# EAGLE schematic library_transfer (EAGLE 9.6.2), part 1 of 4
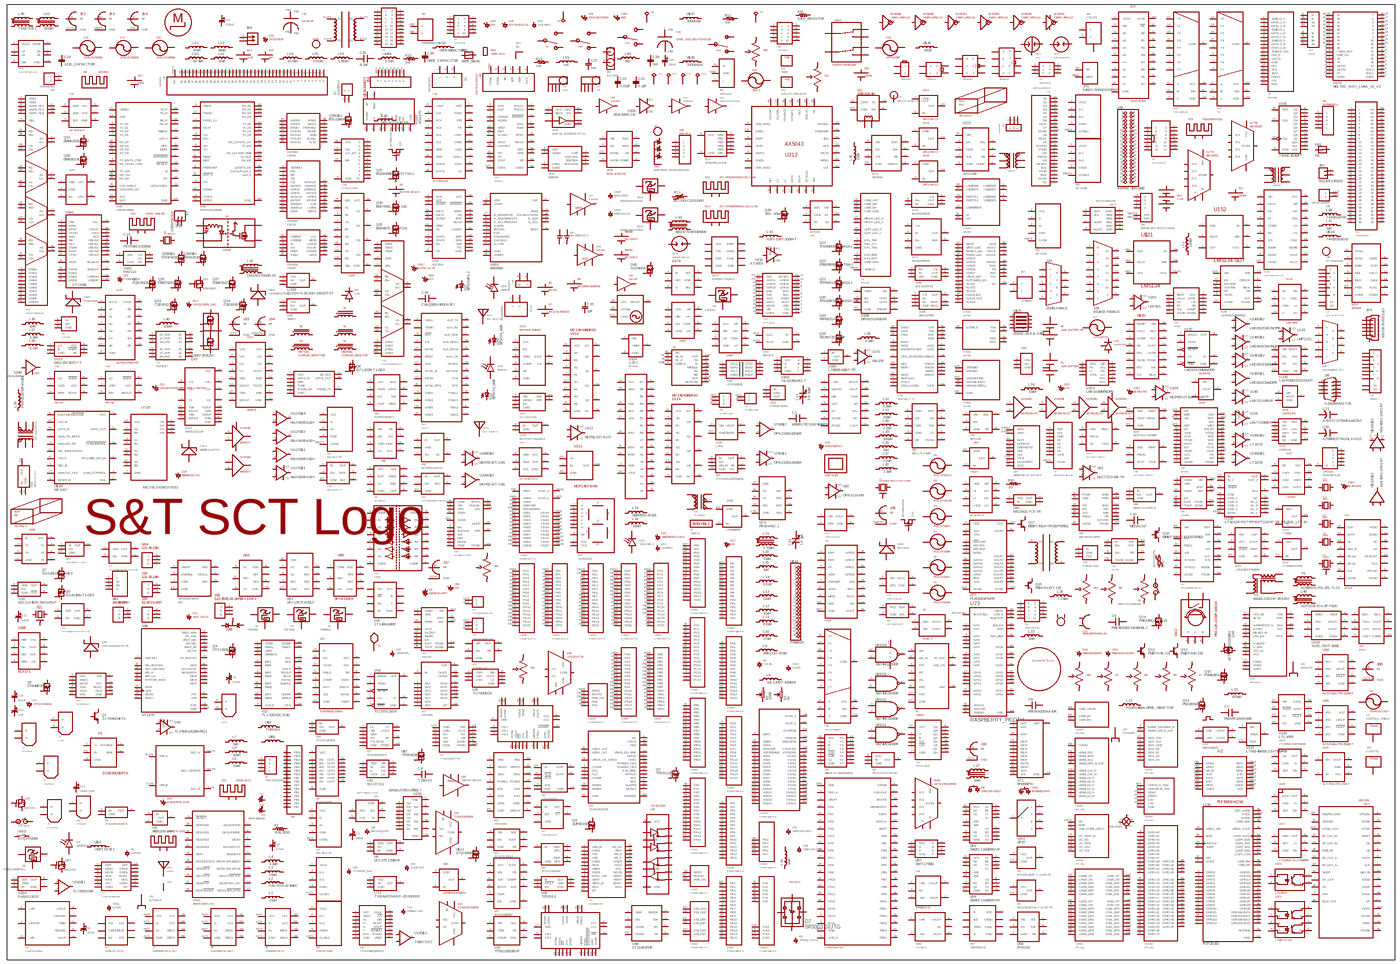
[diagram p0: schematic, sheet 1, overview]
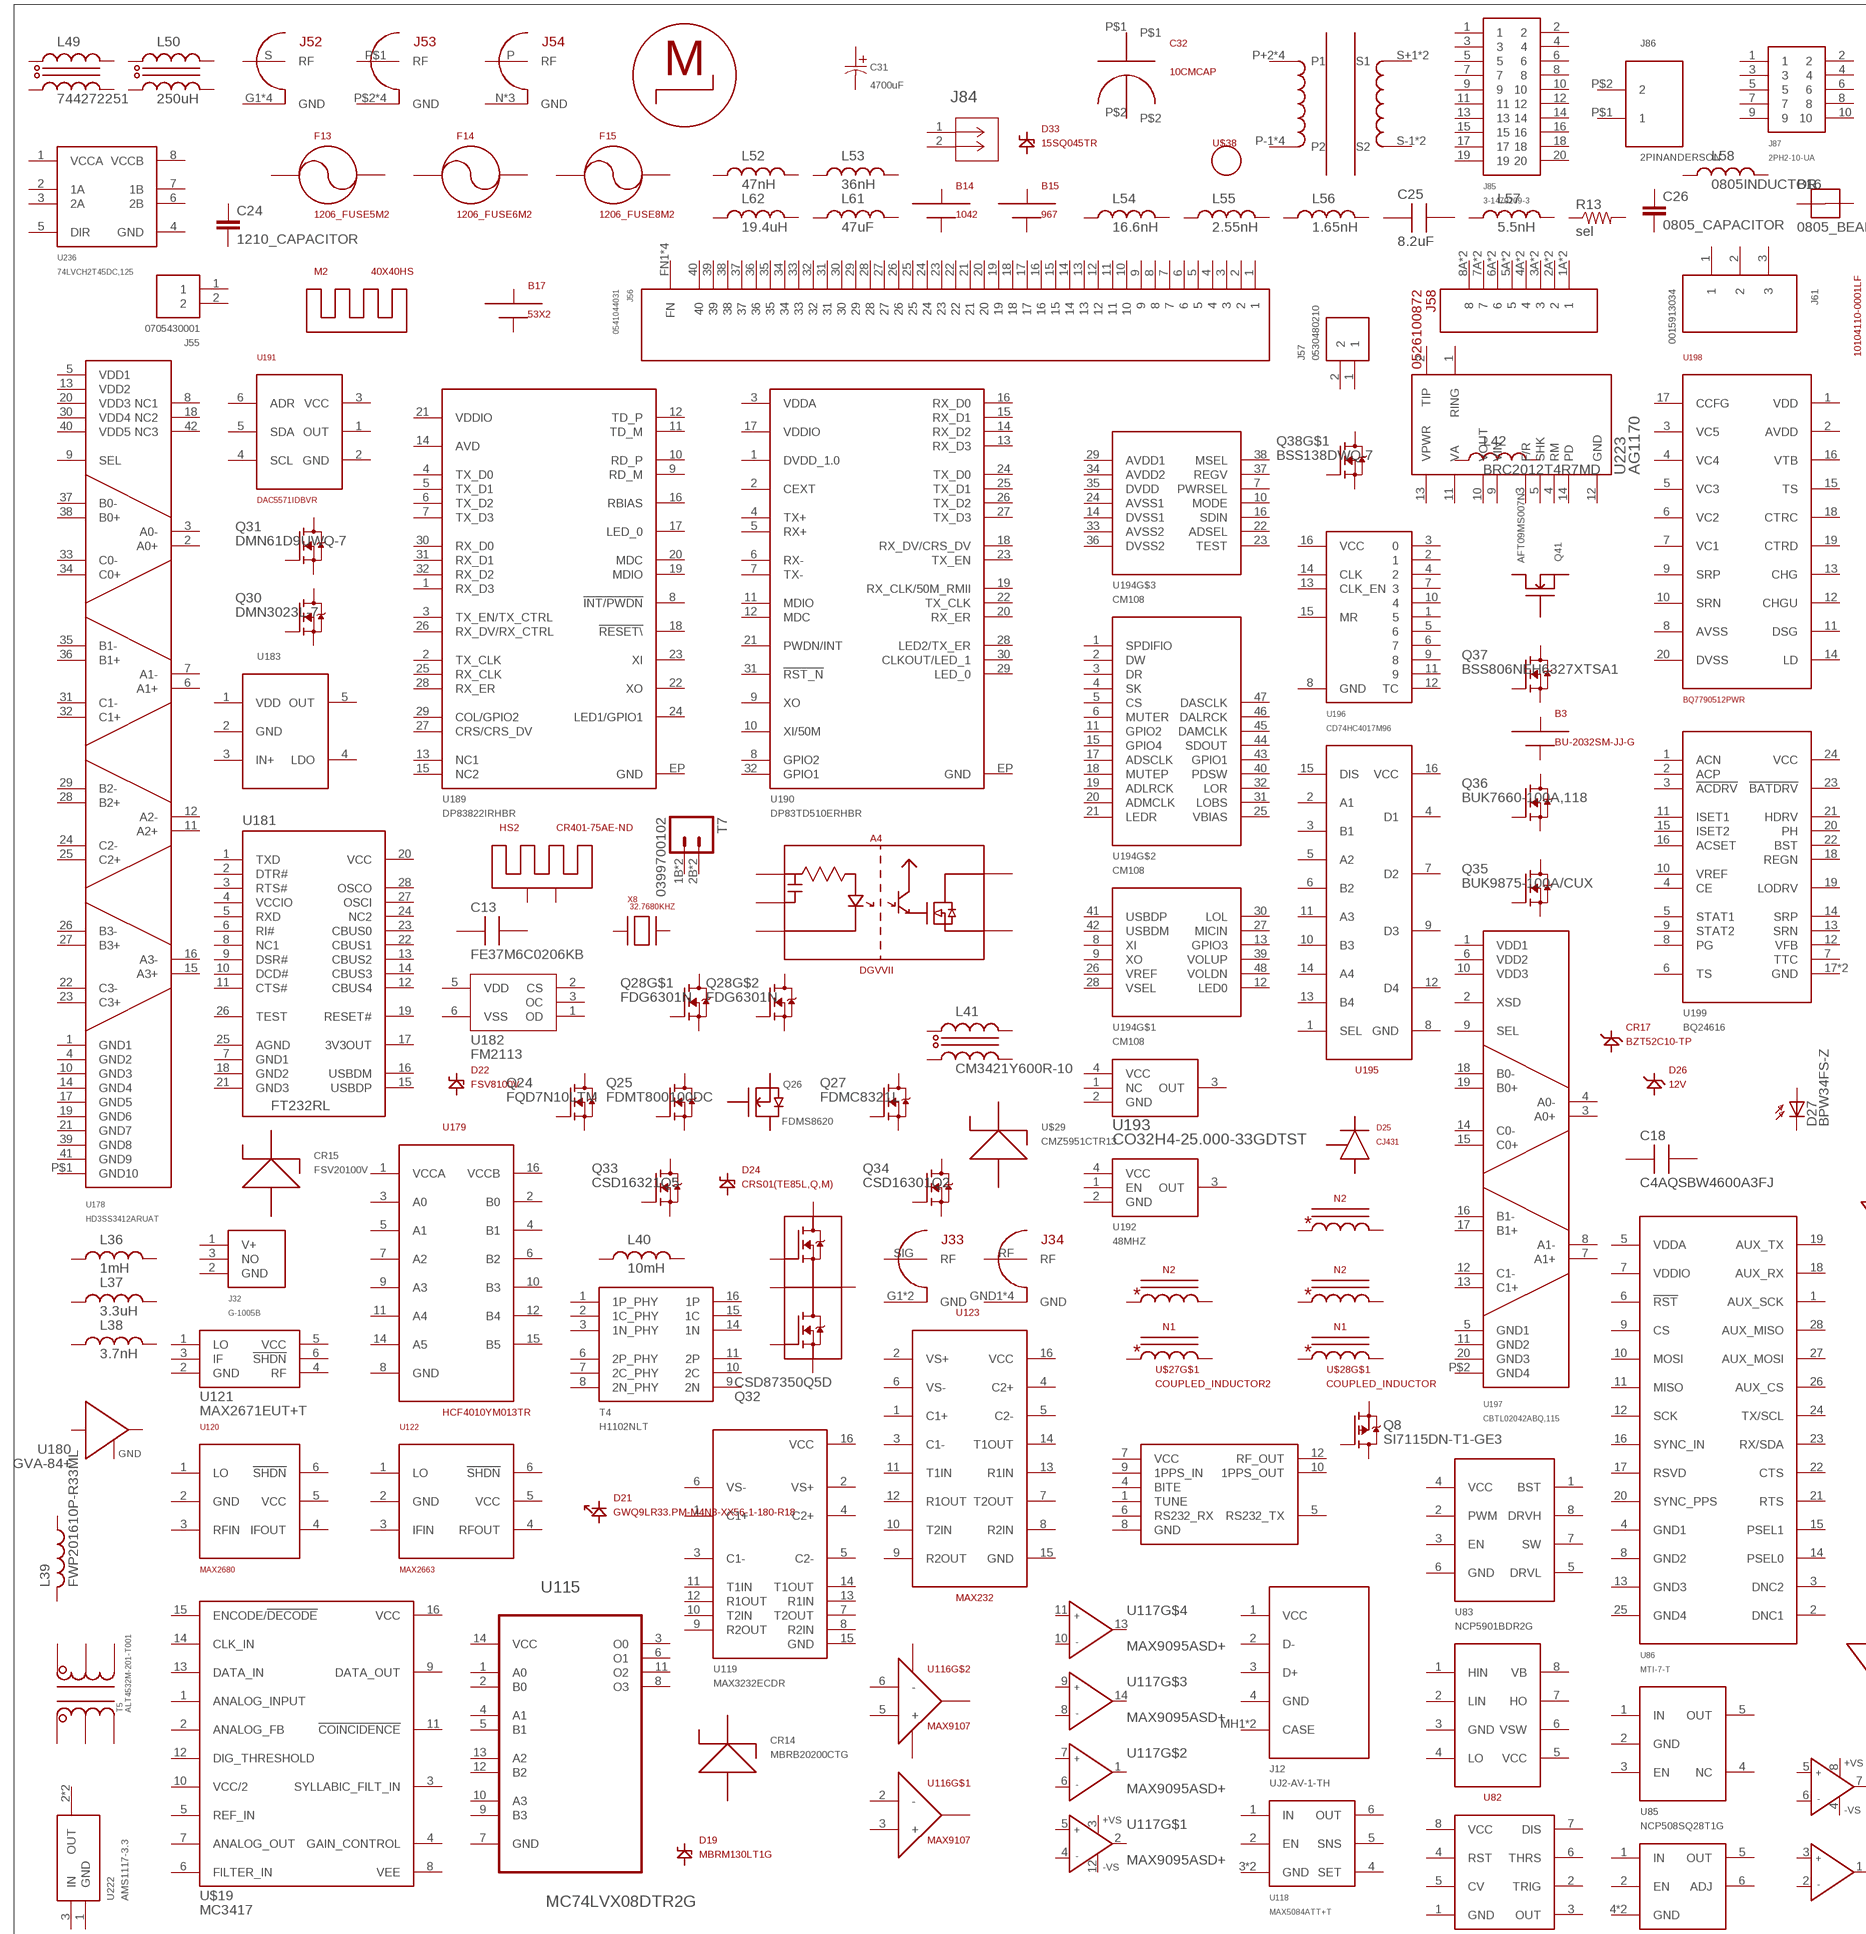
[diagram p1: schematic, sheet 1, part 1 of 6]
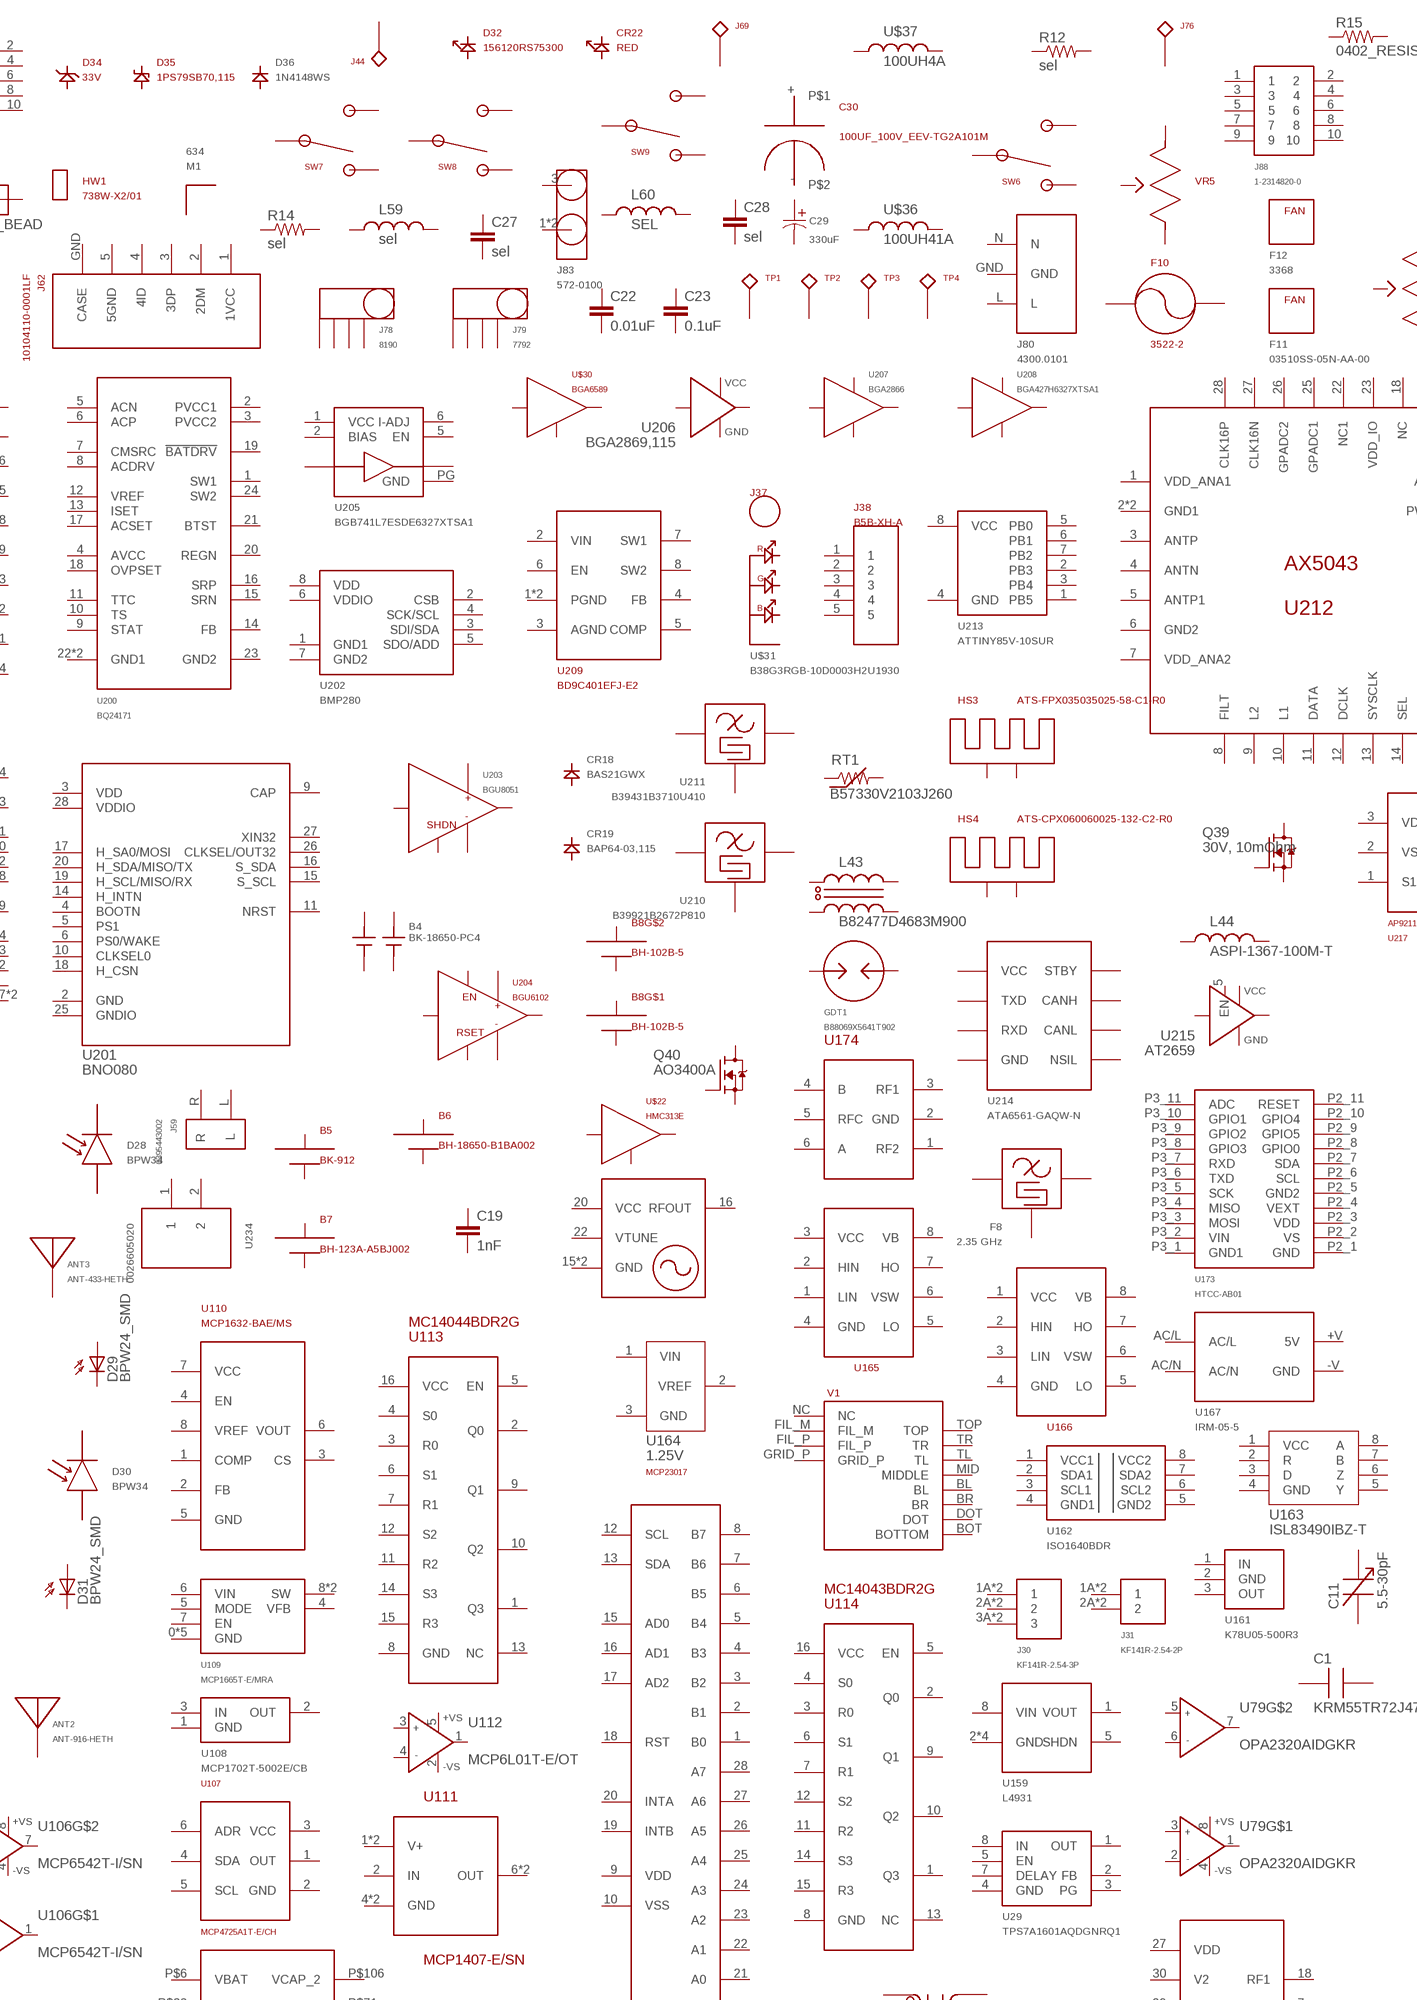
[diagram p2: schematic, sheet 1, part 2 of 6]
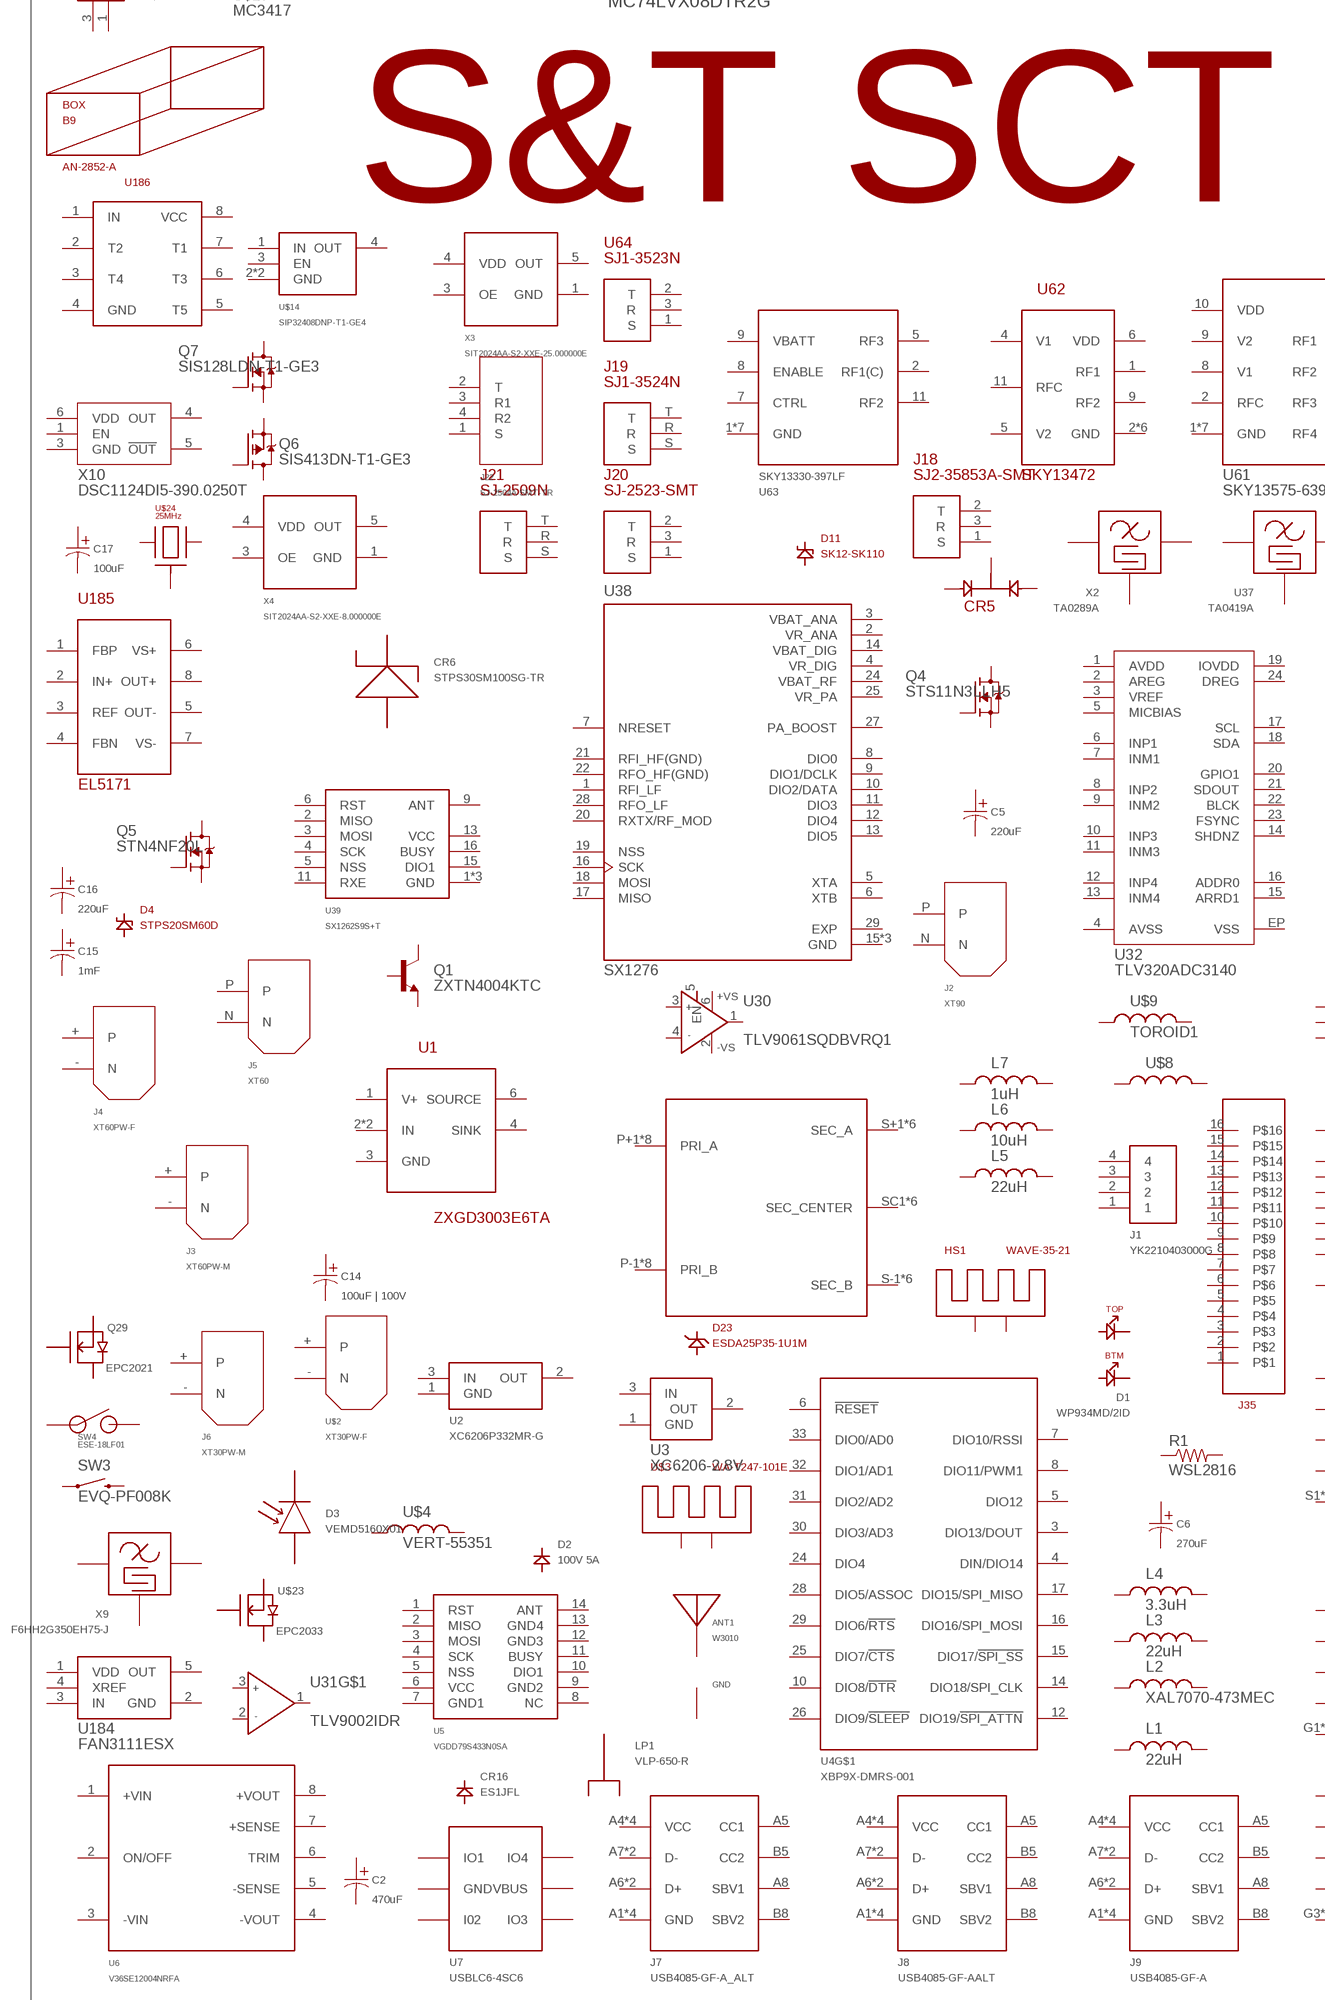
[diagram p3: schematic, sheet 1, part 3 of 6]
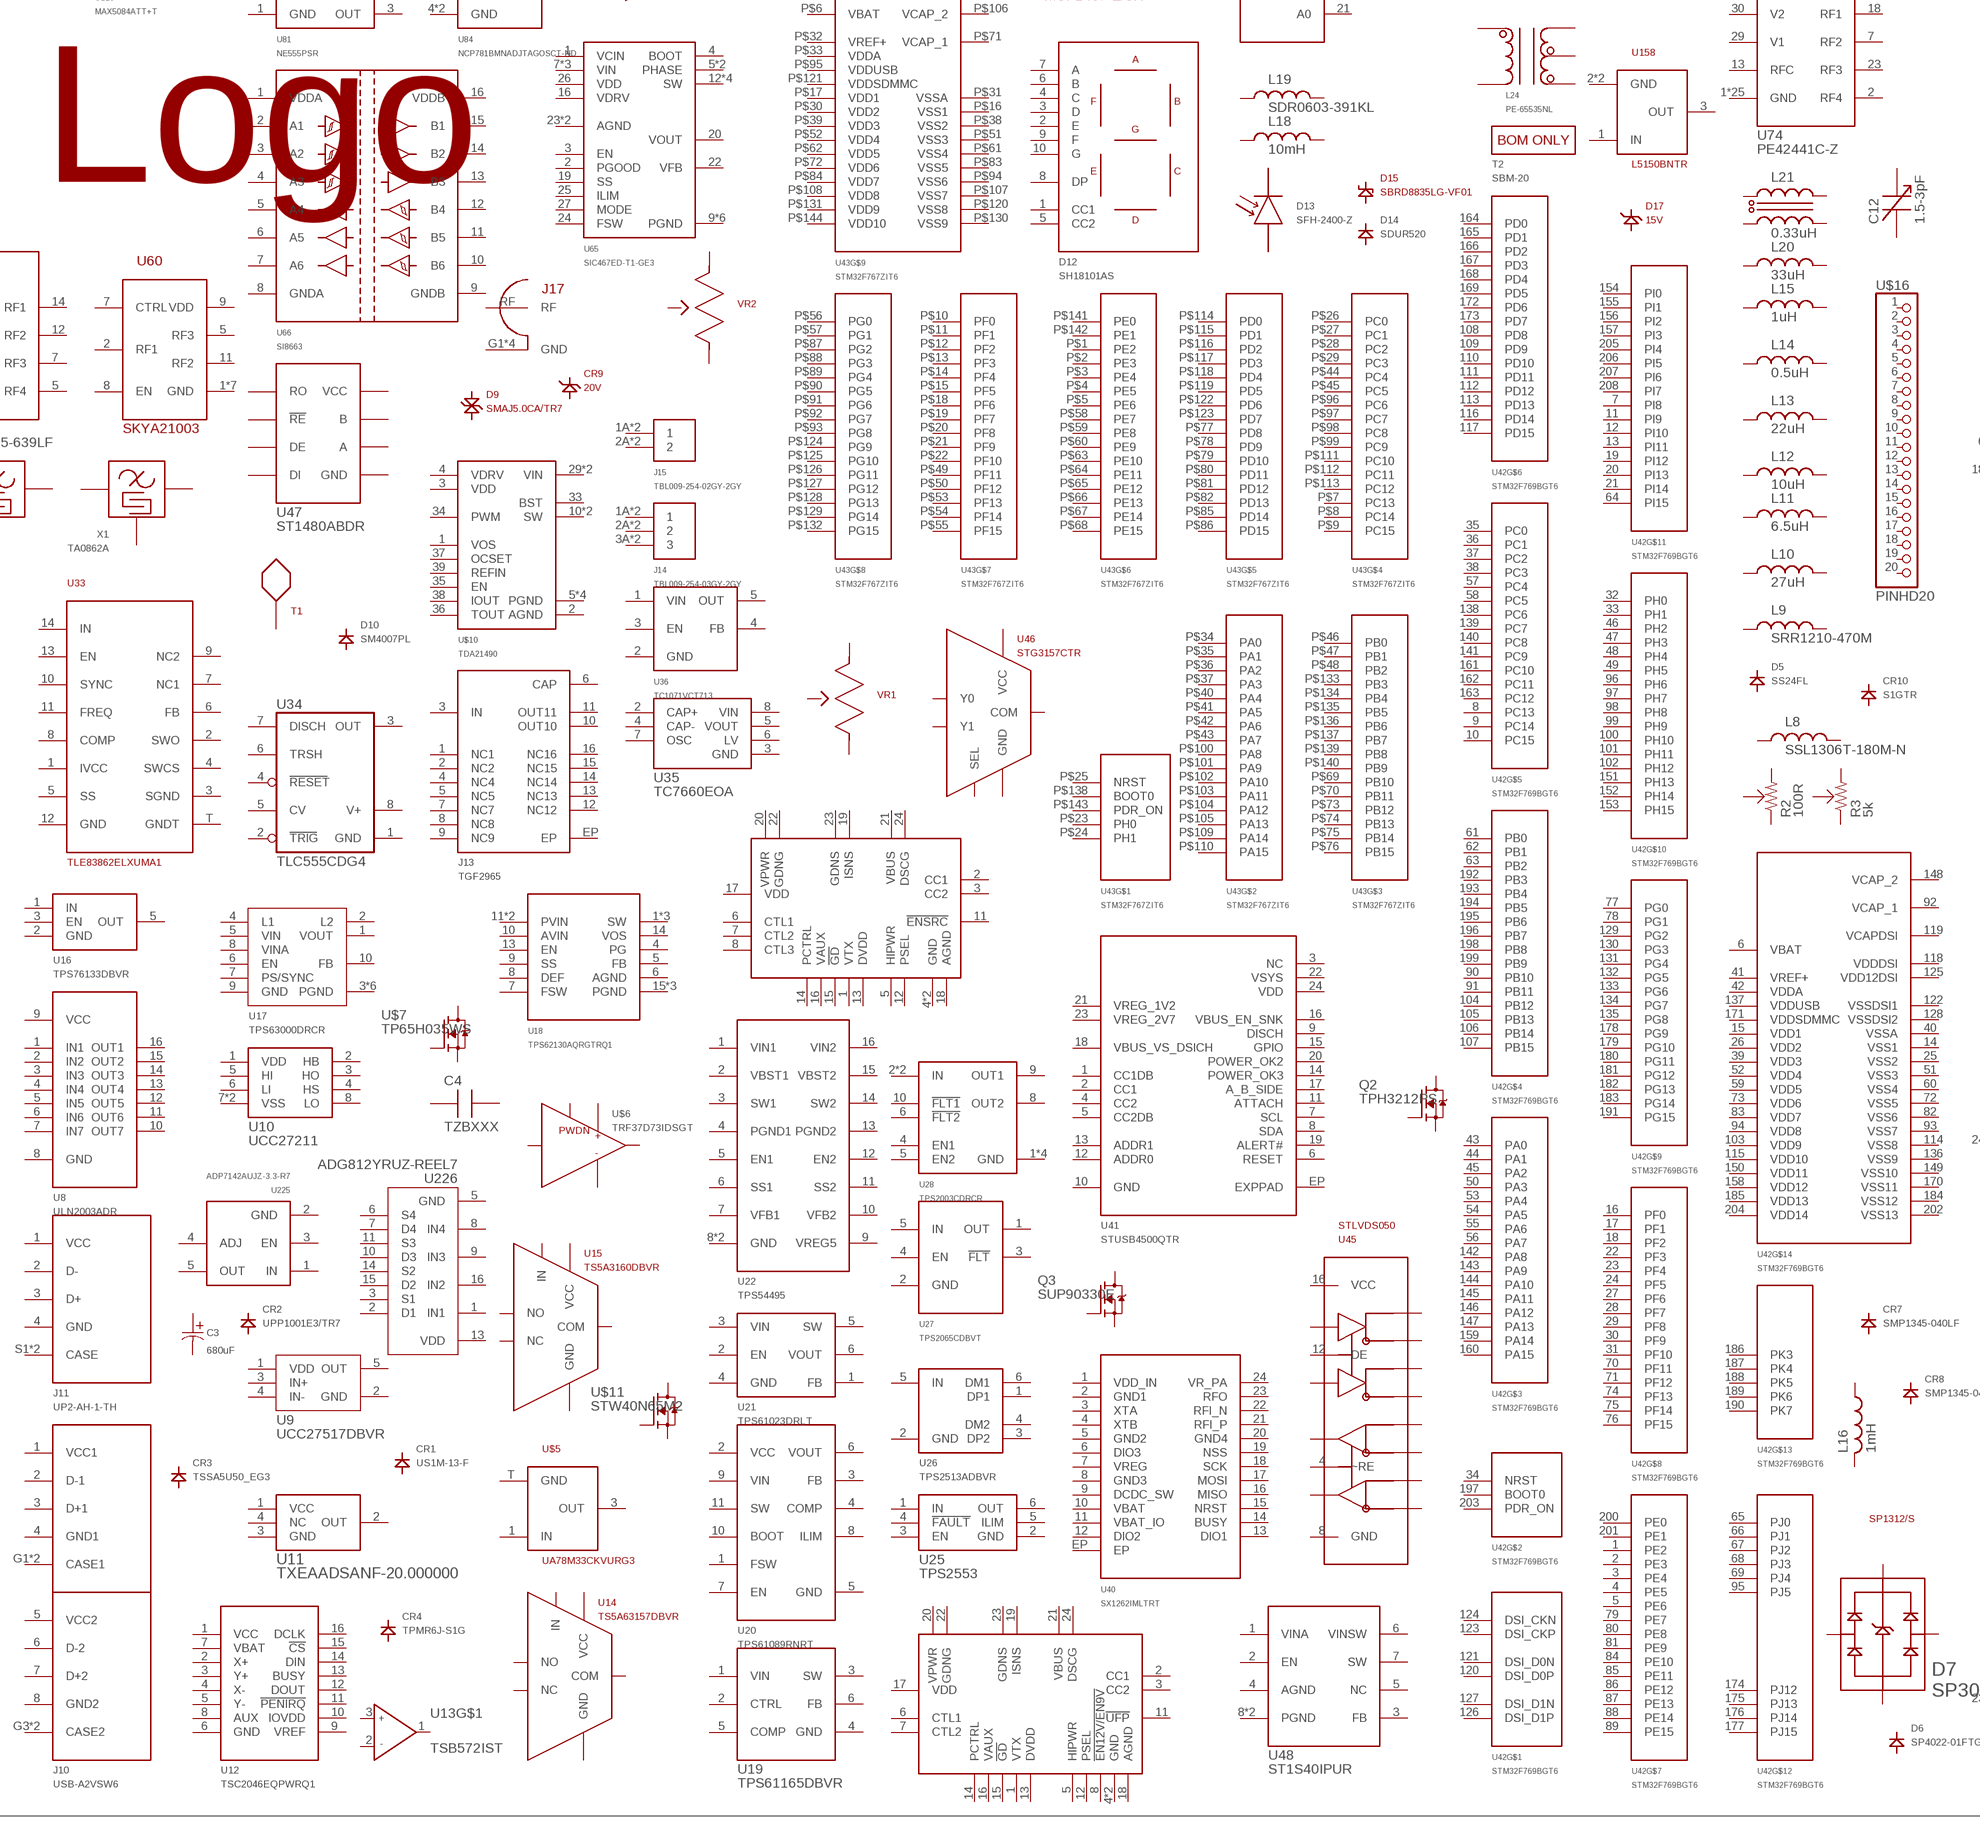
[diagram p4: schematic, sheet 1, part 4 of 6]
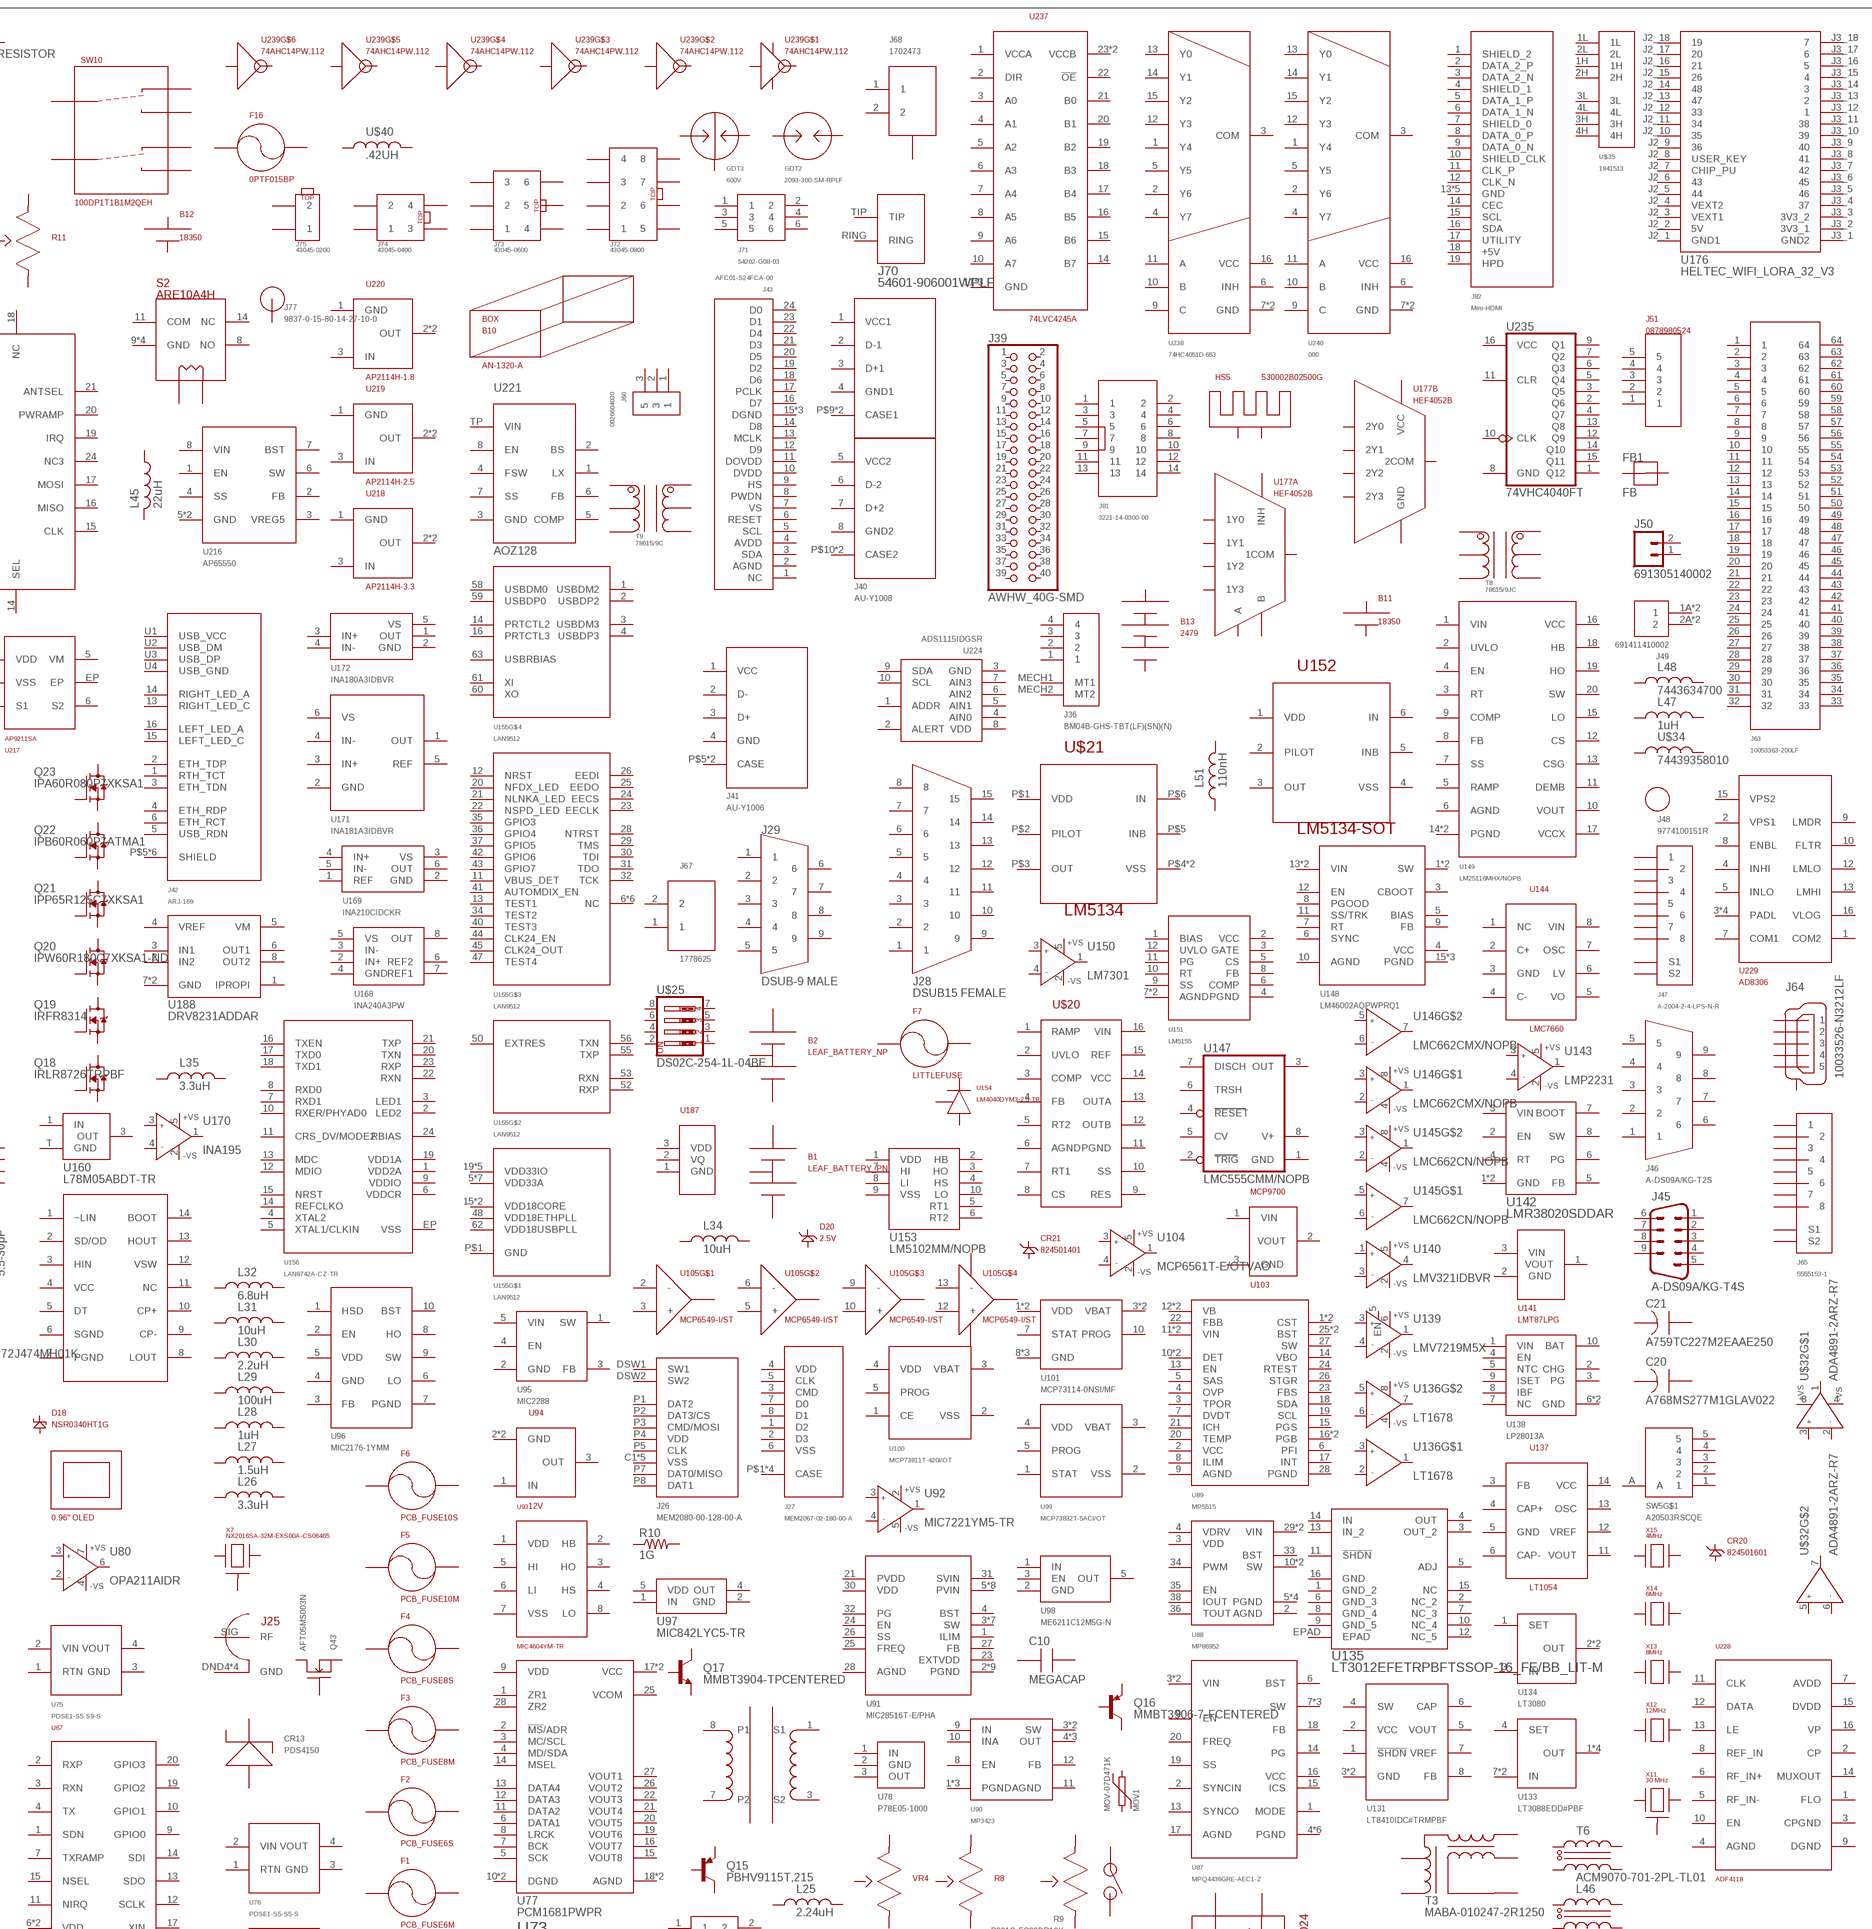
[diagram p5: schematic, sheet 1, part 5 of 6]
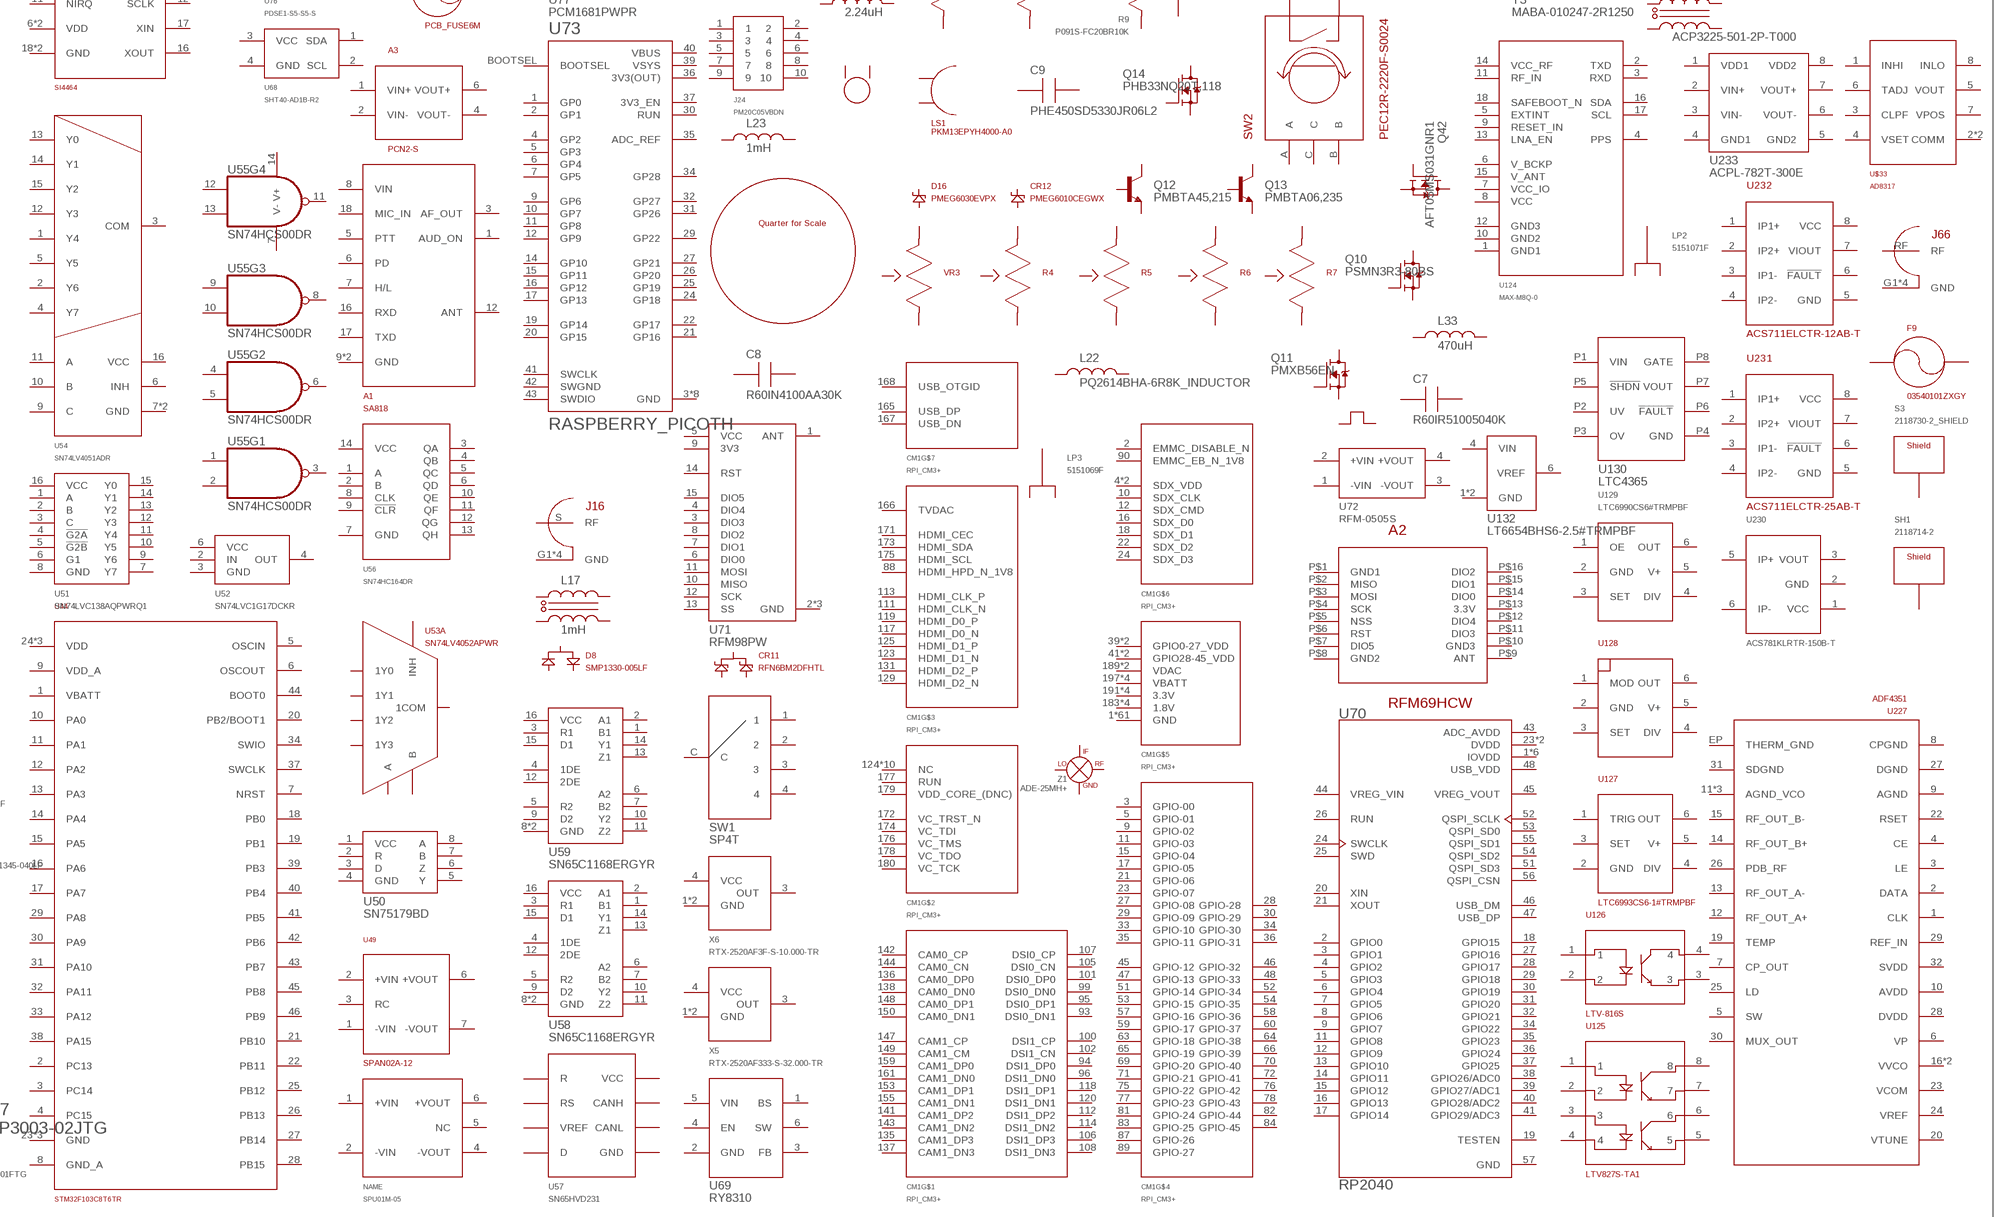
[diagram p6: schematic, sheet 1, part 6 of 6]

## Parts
A1  SA818  [SA818]
A2  RFM69HCW  [RFM69HCW]
A3  PCN2-S  [PCN2-S]
A4  DGVVII  [DGD8]
ANT1  W3010  [W3010]
ANT2  ANT-916-HETH  [ANT-916-HETH]
ANT3  ANT-433-HETH  [ANT-433-HETH]
B1  LEAF_BATTERY_PN  [LEAF_BATTERY]
B2  LEAF_BATTERY_NP  [LEAF_BATTERY]
B3  BU-2032SM-JJ-G  [BU-2032SM-JJ-G]
B4  BK-18650-PC4  [2-18650]
B5  BK-912  [BK-912]
B6  BH-18650-B1BA002  [18650]
B7  BH-123A-A5BJ002  [BH-123A-A5BJ002]
B8  BH-102B-5  [BH-102B-5]
B9  AN-2852-A  [HBAN2852]
B10  AN-1320-A  [HBAN1320]
B11  18350  [18350]
B12  18350  [18350]
B13  2479  [3AAA]
B14  1042  [1042]
B15  967  [967]
B16  0805_BEAD  [0805]
B17  53X2  [53X2]
C1  KRM55TR72J474MH01K  [KRM55TR72J474MH01K]
C2  470uF  UVR2A471MHD  [CAP-7.5-16]
C3  680uF  UCL1E681MNL1GS  [UCL1E681MNL1GS]
C4  TZBXXX  [TZB]
C5  220uF  T521X227M016ATE035  [2917]
C6  270uF  SLPX271M200A1P3  [CAP-10-22MM]
C7  R60IR51005040K  [R60IR51005040K]
C8  R60IN4100AA30K  [R60IN4100AA30K]
C9  PHE450SD5330JR06L2  [PHE450SD5330JR06L2]
C10  MEGACAP  [MEGACAP45]
C11  5.5-30pF  JZ300  [JZ300]
C12  1.5-3pF  JZ030  [JZ300]
C13  FE37M6C0206KB  [FE37M6C0206KB]
C14  100uF | 100V  EMVY101ARA101MKE0S  [13X13CAP]
C15  1mF  EKYB630ELL102ML25S  [CAP-7.5-16]
C16  220uF  EEE-TG1E221UP  [EEE-TG1E221UP]
C17  100uF  EEE-HC1C101XP  [6.6X6.6CAP]
C18  C4AQSBW4600A3FJ  [C4AQBF]
C19  1nF  B32529C6102K289  [5MM_FILM]
C20  A768MS277M1GLAV022  [A768]
C21  A759TC227M2EAAE250  [A759_22X45]
C22  0.01uF  06035C103KAT4A  [0603]
C23  0.1uF  06033C104KAT4A  [0603]
C24  1210_CAPACITOR  [1210]
C25  8.2uF  825MMR250K  [1.083FILM]
C26  0805_CAPACITOR  [0805]
C27  sel  0603_CAPACITOR  [0603]
C28  sel  0402_CAPACITOR  [0402_INDUCTOR]
C29  330uF  200KXW330MEFC16X35  [CAP-7.5-16]
C30  100UF_100V_EEV-TG2A101M  [CPOL17X17]
C31  4700uF  25PK4700MEFC16X25  [25PK4700MEFC16X25]
C32  10CMCAP  [10CMCAP]
CM1  RPI_CM3+  [DDR2_SODIMM]
CR1  US1M-13-F  [DO-214AC]
CR2  UPP1001E3/TR7  [DO-216]
CR3  TSSA5U50_EG3  [DO-214AC]
CR4  TPMR6J-S1G  [TO-277]
CR5  STPSC20H12CWL  [TO-247]
CR6  STPS30SM100SG-TR  [D2PAK]
CR7  SMP1345-040LF  [SOD882]
CR8  SMP1345-040LF  [SOD882]
CR9  20V  SMAJ20A  [DO-214AC]
CR10  S1GTR  [DO-214AC]
CR11  RFN6BM2DFHTL  [TO-252]
CR12  PMEG6010CEGWX  [SOD123(AK)]
CR13  PDS4150  [POWERD15]
CR14  MBRB20200CTG  [D2PAK]
CR15  FSV20100V  [TO-277]
CR16  ES1JFL  [SOD123(AK)]
CR17  BZT52C10-TP  [SOD123(AK)]
CR18  BAS21GWX  [SOD123]
CR19  BAP64-03,115  [SOD323]
CR20  824501601  [DO-214AC]
CR21  824501401  [DO-214AC]
CR22  RED  150060RS75000  [0603_DIODE]
D1  WP934MD/2ID  [WP934MD/2ID]
D2  100V 5A  VSSAF510-M3/H  [DO-221AC]
D3  VEMD5160X01  [VEMD5160X01]
D4  STPS20SM60D  [TO-220-2]
D5  SS24FL  [SOD123(AK)]
D6  SP4022-01FTG  [SOD323]
D7  SP3003-02JTG  [SC-70-5]
D8  SMP1330-005LF  [SOT23-3]
D9  SMAJ5.0CA/TR7  [DO-214AC_NO_POL]
D10  SM4007PL  [SOD123(AK)]
D11  SK12-SK110  [SMB]
D12  SH18101AS  [SH18101AS]
D13  SFH-2400-Z  [SFH2400]
D14  SDUR520  [TO-220-2]
D15  SBRD8835LG-VF01  [TO-252]
D16  PMEG6030EVPX  [SOD128]
D17  15V  PDZ15BGWX  [SOD123(AK)]
D18  NSR0340HT1G  [SOD323]
D19  MBRM130LT1G  [DO-216]
D20  2.5V  LM4040  [SOT23-3]
D21  GWQ9LR33.PM-M4N3-XX56-1-180-R18  [Q9LR33]
D22  FSV8100V  [TO-277]
D23  ESDA25P35-1U1M  [1610]
D24  CRS01(TE85L,Q,M)  [SOD123(AK)]
D25  CJ431  [SOT23-3_CENTERED]
D26  12V  BZX84C12LT1G  [SOT23-3]
D27  BPW34FS-Z  [BPW34_SMD]
D28  BPW34  [BPW34]
D29  BPW24_SMD  [BPX65]
D30  BPW34  [BPW34]
D31  BPW24_SMD  [BPX65]
D32  156120RS75300  [1206_REV]
D33  15SQ045TR  [LONG_DIODE]
D34  33V  1SMA5937BT3GDO-  [DO-214AC]
D35  1PS79SB70,115  [SOD-523]
D36  1N4148WS  [SOD323]
F1  PCB_FUSE6M  [1206_FUSE_6M]
F2  PCB_FUSE6S  [1206_FUSE_6S]
F3  PCB_FUSE8M  [1206_FUSE_8M]
F4  PCB_FUSE8S  [1206_FUSE_8S]
F5  PCB_FUSE10M  [1206_FUSE_10M]
F6  PCB_FUSE10S  [1206_FUSE_10S]
F7  LITTLEFUSE  [LITTLEFUSE]
F8  2.35 GHz  B39232B9628P810  [B9628]
F9  03540101ZXGY  [1.25IN_FUSE]
F10  3522-2  [FUSE_SOCKET]
F11  03510SS-05N-AA-00  [35MMFAN]
F12  3368  [30MMFAN]
F13  1206_FUSE5M2  [1206_FUSE_5M2]
F14  1206_FUSE6M2  [1206_FUSE_6M2]
F15  1206_FUSE8M2  [1206_FUSE_8M2]
F16  0PTF015BP  [0PTF015BP]
FB1  FB  2518065007Y6  [1806]
GDT1  B88069X5641T902  [ES1200XSMD]
GDT2  2093-300-SM-RPLF  [2093-300-SM-RPLF]
GDT3  600V  2036-60-SM-RPLF  [2036_GDT]
HS1  WAVE-35-21  [WAVE-35-21]
HS2  CR401-75AE-ND  [CR401]
HS3  ATS-FPX035035025-58-C1-R0  [ATS-FPX035035025-58-C1-R0]
HS4  ATS-CPX060060025-132-C2-R0  [ATS-CPX060060025-132-C2-R0]
HS5  530002B02500G  [530002]
HW1  738W-X2/01  [738W-X2/01]
J1  YK2210403000G  [YK2210403000G]
J2  XT90  [XT90]
J3  XT60PW-M  [XT-60-PW-M]
J4  XT60PW-F  [XT-60-PW-F]
J5  XT60  [XT60]
J6  XT30PW-M  [XT30PW-M]
J7  USB4085-GF-A_ALT  [USBC]
J8  USB4085-GF-AALT  [USBC2]
J9  USB4085-GF-A  [USBC]
J10  USB-A2VSW6  [VERT2XUSB]
J11  UP2-AH-1-TH  [UP2-AH-1-TH]
J12  UJ2-AV-1-TH  [UJ2-AV-1-TH]
J13  TGF2965  [216-5205-01]
J14  TBL009-254-03GY-2GY  [TBL009-254-03GY-2GY]
J15  TBL009-254-02GY-2GY  [TBL009-254-02GY-2GY]
J16  SMA_0732511150  [WIDE_SMA]
J17  SMAFSTJ.B.HT  [SMA]
J18  SJ2-35853A-SMT  [SJ2]
J19  SJ1-3524N  [3.5MM_TRS]
J20  SJ-2523-SMT  [SJ]
J21  SJ-2509N  [2.5MM_TRS]
J22  SJ-2504A-SMT-TR  [SJ-2504A-SMT-TR]
J23  RENAME  [ROINT]
J24  PM20C05VBDN  [PM20C05VBDN]
J25  PCB.SMAFSTJ.B.HT  [SMA_SMD_VERT]
J26  MEM2080-00-128-00-A  [MEM2080]
J27  MEM2067-02-180-00-A  [MICRO_SD]
J28  DSUB15 FEMALE  LD15S24A4GV00LF  [DSUB15_VERT]
J29  DSUB-9 MALE  LD09P24A4GV00LF  [DSUB9_VERT]
J30  KF141R-2.54-3P  [KF141R-2.54-3P]
J31  KF141R-2.54-2P  [KF141R-2.54-2P]
J32  G-1005B  [G-1005B]
J33  CONUFL001-SMD  [U.FL]
J34  CON-SMA-EDGE-S  [CON-SMA-EDGE-S]
J35  BMIV3  [BMIV16]
J36  BM04B-GHS-TBT(LF)(SN)(N)  [BM04B-GHS-TBT(LF)(SN)(N)]
J37  BANANA  [BANANA]
J38  B5B-XH-A  [B5B-XH-A]
J39  AWHW_40G-SMD  [SMD40]
J40  AU-Y1008  [AU-Y1008]
J41  AU-Y1006  [USBA_SMD]
J42  ARJ-169  [ARJ-169]
J43  AFC01-S24FCA-00  [AFC01-S24FCA-00]
J44  16008-83-4810  [16008-83-4810]
J45  A-DS09A/KG-T4S  [DB9]
J46  A-DS09A/KG-T2S  [A-DS09A/KG-T2S]
J47  A-2004-2-4-LPS-N-R  [A-2004-2-4-LPS-N-R]
J48  9774100151R  [9774100151R]
J49  691411410002  [691411410002]
J50  691305140002  [691305140002]
J51  0878980524  [5-SMT-HEADER]
J52  0733910070  [CONREVSMA008-G]
J53  0731711900  [0731711900]
J54  0731385033  [0731385033]
J55  0705430001  [SL2]
J56  0541044031  [54104-4031]
J57  0530480210  [0530480210]
J58  0526100872  [0526100872]
J59  0395443002  [0395443002]
J60  0026604030  [0026604030]
J61  0015913034  [3-SL_SMT]
J62  10104110-0001LF  [MICRO_USB]
J63  10053363-200LF  [10053363-200LF]
J64  10033526-N3212LF  [MINI_USB]
J65  5555153-1  [5555153-1]
J66  5413631-1  [5413631-1]
J67  1778625  [1778625]
J68  1702473  [1702473]
J69  01010002Z  [01010002Z]
J70  54601-906001WPLF  [54601-906001WPLF]
J71  54202-G08-03  [6-SMT-HEADER]
J72  43045-0800  [43045-0800]
J73  43045-0600  [43045-0600]
J74  43045-0400  [43045-0400]
J75  43045-0200  [43045-0200]
J76  16008-83-4810  [16008-83-4810]
J77  9837-0-15-80-14-27-10-0  [9837]
J78  8190  [7781]
J79  7792  [7792]
J80  4300.0101  [4300.0101]
J81  3221-14-0300-00  [3221-14-0300-00]
J82  Mini-HDMI  2001-1-2-21-00-BK  [MINI_HDMI]
J83  572-0100  [572-0100]
J84  24.243.1  [CONN_24.243_MTC]
J85  3-1470209-3  [10X2_2MM]
J86  2PINANDERSON  [APP]
J87  2PH2-10-UA  [2PH2-10-UA]
J88  1-2314820-0  [5X2_2MM]
L1  22uH  XAL8080-223MED  [XAL8080]
L2  XAL7070-473MEC  [XAL7070]
L3  22uH  XAL6060-223MEC  [XAL6060]
L4  3.3uH  XAL4030-332  [COILCRAFT_XAL4030]
L5  22uH  TMPC0603H-220MG-D  [TMPC0603H]
L6  10uH  TMPC0603H-100MG-D  [TMPC0603H]
L7  1uH  TMPC0603H-1R0MG-D  [TMPC0603H]
L8  SSL1306T-180M-N  [SSL1306T]
L9  SRR1210-470M  [DR125]
L10  27uH  SRR1208-270ML  [SRR1208]
L11  6.5uH  SRR1208-6R5ML  [SRR1208]
L12  10uH  SRP1265C-100M  [SRP1265]
L13  22uH  SRP1265A-220M  [SRP1265]
L14  0.5uH  SRN8040TA-R50Y  [SRN8040]
L15  1uH  SRN8040TA-1R0Y  [SRN8040]
L16  1mH  SNR5040TYD102M  [SNR5040]
L17  1mH  SMCM090605-102  [SMCM090605]
L18  10mH  SDR1005-103KL  [SDR1005]
L19  SDR0603-391KL  [SDR0603]
L20  33uH  SDR0403-330KL  [SDR0403]
L21  0.33uH  SDCW2520S-2-601TF  [SDCW2520]
L22  PQ2614BHA-6R8K_INDUCTOR  [PQ2614BHA-6R8K]
L23  1mH  PM2120-102K-RC  [PM2120]
L24  PE-65535NL  [PE-65535NL]
L25  2.24uH  PA0489LNL  [PA0489LNL]
L26  3.3uH  NS10165T3R3NNA  [NS10165]
L27  1.5uH  NRS8030T1R5NJGJ  [NRS8030]
L28  1uH  NRS8030T1R0NJGJ  [NRS8030]
L29  100uH  NR6028T101M  [NR6028]
L30  2.2uH  NR6028T2R2N  [NR6028]
L31  10uH  NR6028  [NR6028]
L32  6.8uH  NR6020T6R8N  [NR6028]
L33  470uH  MSRH104R-471MT  [MSRH104R]
L34  10uH  LHL08TB100K  [LHL08TB100K]
L35  3.3uH  IHLP2020CZER3R3M11  [IHLP-2020CZ-11]
L36  1mH  HCTI-1000-2.4  [HCTI-1000-2.4]
L37  3.3uH  HCM1307-3R3-R  [HCM1307]
L38  3.7nH  GA3092-AL  [GA3092]
L39  FWP201610P-R33ML  [0806]
L40  10mH  FNR8065S103MT  [FNR8065S]
L41  CM3421Y600R-10  [CM3421Y600R-10]
L42  BRC2012T4R7MD  [0805]
L43  B82477D4683M900  [B82477D4683M900]
L44  ASPI-1367-100M-T  [ASPI-1367-100M-T]
L45  22uH  APW12A10  [APW12A10]
L46  ACP3225-501-2P-T000  [3225]
L47  1uH  74438357010  [74438357010]
L48  7443634700  [WE-HCF]
L49  744272251  [744272221]
L50  250uH  744272221  [744272221]
L51  110nH  2222SQ-111  [2222SQ-111]
L52  47nH  1111SQ-47N  [1111SQ-47N]
L53  36nH  1111SQ-36NGEC  [111SQ-36N]
L54  16.6nH  0908SQ--17NGLC  [COILCRAFT_0908SQ--17NGLC]
L55  2.55nH  0906--3JLC  [COILCRAFT_0906]
L56  1.65nH  0906--2KLC  [COILCRAFT_0906]
L57  5.5nH  0806SQ--5N5GLC  [COILCRAFT_0806SQ--5N5GLC]
L58  0805INDUCTOR  [0805]
L59  sel  0603_INDUCTOR  [0603]
L60  SEL  0402_INDUCTOR  [0402_INDUCTOR]
L61  47uF  60B473C  [6000BINDUCTOR]
L62  19.4uH  60A193C  [6000AINDUCTOR]
LP1  VLP-650-R  [VLP-XXX-R]
LP2  5151071F  [5151071F]
LP3  5151069F  [5151069F]
LS1  PKM13EPYH4000-A0  [PKM13EPYH4000-A0]
M1  634  [634]
M2  40X40HS  [40X40HS]
MOV1  MOV-07D471K  [MOV-07D471K]
Q1  ZXTN4004KTC  [TO-252]
Q2  TPH3212PS  [TO-220]
Q3  SUP90330E  [TO-220]
Q4  STS11N3LLH5  [SOIC8]
Q5  STN4NF20L  [SOT223]
Q6  SIS413DN-T1-GE3  [POWERPAK_1212-8]
Q7  SIS128LDN-T1-GE3  [POWERPAK_SO-8]
Q8  SI7115DN-T1-GE3  [POWERPAK_1212-8]
Q9  QUARTER  [QUARTER]
Q10  PSMN3R3-80BS  [D2PAK]
Q11  PMXB56EN  [DFN1010D3]
Q12  PMBTA45,215  [SOT23-3]
Q13  PMBTA06,235  [SOT23-3]
Q14  PHB33NQ20T,118  [D2PAK]
Q15  PBHV9115T,215  [SOT23-3]
Q16  MMBT3906-7-FCENTERED  [SOT23-3_CENTERED]
Q17  MMBT3904-TPCENTERED  [SOT23-3_CENTERED]
Q18  IRLR8726TRPBF  [TO-252]
Q19  IRFR8314  IRFR8314TRPBF  [TO-252]
Q20  IPW60R180C7XKSA1-ND  [TO-247]
Q21  IPP65R125C7XKSA1  [TO-220]
Q22  IPB60R060P7ATMA1  [D2PAK]
Q23  IPA60R080P7XKSA1  [TO-220]
Q24  FQD7N10LTM  [TO-252]
Q25  FDMT800100DC  [8-POWERVDFN]
Q26  FDMS8620  [POWER56]
Q27  FDMC8321L  [POWER33]
Q28  FDG6301N  [SC-70]
Q29  EPC2021  [EPC30]
Q30  DMN3023L-7  [SOT23-3]
Q31  DMN61D9UWQ-7  [SOT-323]
Q32  CSD87350Q5D  [8LSON]
Q33  CSD16321Q5  [8-POWERTDFN]
Q34  CSD16301Q2  [2X2SON]
Q35  BUK9875-100A/CUX  [SOT223]
Q36  BUK7660-100A,118  [7109D2PAK]
Q37  BSS806NEH6327XTSA1  [SOT23-3_CENTERED]
Q38  BSS138DWQ-7  [SOT-363]
Q39  30V, 10mOhm  AO4576  [SOIC8]
Q40  AO3400A  [SOT23-3_CENTERED]
Q41  AFT09MS007N  [PLD-1.5W]
Q42  AFT05MS031GNR1  [TO-270-2-GULL]
Q43  AFT05MS003N  [SOT-89A]
R1  WSL2816  [2816]
R2  100R  ST-4ETB101  [ST-4]
R3  5k  ST-4ETA502  [SMDPOT]
R4  10k  PTV09A-4025F-A103  [PTV09]
R5  PTV09A-4020F-B102  [PTV09]
R6  PTV09A-4020F-A504  [PTV09]
R7  PTV09A-2020F-B103  [PTV09R]
R8  P160KN  [P160KN]
R9  P091S-FC20BR10K  [P091S]
R10  1G  MHR0317SA108F70  [MHR0317_SMD]
R11  10  3361P-1-100GLF  [3361P]
R12  sel  2512_RESISTOR  [2512]
R13  sel  0805_RESISTOR  [0805]
R14  sel  0603_RESISTOR  [0603]
R15  0402_RESISTOR  [R0402]
RT1  B57330V2103J260  [0603]
S1  SCTLOGO  [SCT]
S2  ARE10A4H  [RFRELAY]
S3  2118730-2_SHIELD  [2118730_SHIELD]
SH1  2118714-2  [2118714-2]
SM1  28BYJ-48  [28-BYJ-48]
SW1  SP4T  RM104772BCB  [RM104772BCB]
SW2  PEC12R-2220F-S0024  [PEC12R]
SW3  EVQ-PF008K  [EVQ-PF008K]
SW4  ESE-18LF01  [ESE-18LF01]
SW5  A20503RSCQE  [A20503RSCQE]
SW6  100SP4T2B4M6RE  [M6SPDT]
SW7  SPDT  100SP1T2B4M6QE  [TOGGLE_RA]
SW8  100SP1T1B4M6RE  [M6SPDT]
SW9  100SP1T1B1M1QEH  [100SP1T1B1M1QEH]
SW10  100DP1T1B1M2QEH  [100DP1T1B1M2QEH]
T1  TEST_POINT  [TEST]
T2  SBM-20  [SBM-20]
T3  MABA-010247-2R1250  [MABA-010247-2R1250]
T4  H1102NLT  [H1102NLT]
T5  ALT4532M-201-T001  [TDK_ALT]
T6  ACM9070-701-2PL-TL01  [ACM9070]
T7  0399700102  [2POS_10.16MM]
T8  78615/9JC  [786]
T9  78615/9C  [786T]
TP1  5011  [5010]
TP2  5010  [5010]
TP3  5002  [5001]
TP4  5001  [5001]
U1  ZXGD3003E6TA  [SOT23-6]
U2  XC6206P332MR-G  [SOT23-3_CENTERED]
U3  XC6206-2.8V  [SOT23-3_CENTERED]
U4  XBP9X-DMRS-001  [SX900]
U5  VGDD79S433N0SA  [VGDD79S433N0SA]
U6  V36SE12004NRFA  [V36SE12004NRFA]
U7  USBLC6-4SC6  [SOT23-6]
U8  ULN2003ADR  [SOIC16]
U9  UCC27517DBVR  [SOT23-5]
U10  UCC27211  [SOIC8_TP]
U11  TXEAADSANF-20.000000  [3.2X2.5_4SMD]
U12  TSC2046EQPWRQ1  [TSSOP16]
U13  TSB572IST  [MSOP-8]
U14  TS5A63157DBVR  [SOT23-6]
U15  TS5A3160DBVR  [SOT23-6]
U16  TPS76133DBVR  [SOT23-5]
U17  TPS63000DRCR  [S-PVSON-N10]
U18  TPS62130AQRGTRQ1  [QFN24-33]
U19  TPS61165DBVR  [SOT23-6]
U20  TPS61089RNRT  [TPS61089RNRT]
U21  TPS61023DRLT  [SOT563]
U22  TPS54495  [TSSOP16-POWER]
U23  TPS25740B  [QFN24-44_TI]
U24  TPS25740  [QFN24-44_TI]
U25  TPS2553  [SOT23-6]
U26  TPS2513ADBVR  [SOT23-6]
U27  TPS2065CDBVT  [SOT23-5]
U28  TPS2003CDRCR  [10-VDFN]
U29  TPS7A1601AQDGNRQ1  [MSOP-8]
U30  TLV9061SQDBVRQ1  [SOT23-6]
U31  TLV9002IDR  [SOIC8]
U32  TLV320ADC3140  [QFN24-55]
U33  TLE83862ELXUMA1  [PG-SSOP-14]
U34  TLC555CDG4  [SOIC8]
U35  TC7660EOA  [SOIC8]
U36  TC1071VCT713  [SOT23-5]
U37  TA0419A  [TAO419]
U38  SX1276  [SX1276]
U39  SX1262S9S+T  [SX1262SXS+T]
U40  SX1262IMLTRT  [QGN24-44]
U41  STUSB4500QTR  [QFN24-44]
U42  STM32F769BGT6  [LQFP208]
U43  STM32F767ZIT6  [LQFP144]
U44  STM32F103C8T6TR  [LQFP48]
U45  STLVDS050  [SO16]
U46  STG3157CTR  [SOT23-6]
U47  ST1480ABDR  [SOIC8]
U48  ST1S40IPUR  [VFQFPN8-4X4]
U49  SPAN02A-12  [SPAN02]
U50  SN75179BD  [SOIC8]
U51  SN74LVC138AQPWRQ1  [TSSOP16]
U52  SN74LVC1G17DCKR  [SC-70]
U53  SN74LV4052APWR  [TSSOP16]
U54  SN74LV4051ADR  [SO16]
U55  SN74HCS00DR  [SOIC-14]
U56  SN74HC164DR  [SOIC-14]
U57  SN65HVD231  [SOIC8]
U58  SN65C1168ERGYR  [PVQFN16]
U59  SN65C1168ERGYR  [PVQFN16]
U60  SKYA21003  [12QFN22]
U61  SKY13575-639LF  [14QFN_1.6X1.6]
U62  SKY13472  [12QFN22]
U63  SKY13330-397LF  [12QFN22]
U64  SJ1-3523N  [SJ1-3523N]
U65  SIC467ED-T1-GE3  [MLP55-27L]
U66  SI8663  SI8663BB-B-IU  [SOIC16W]
U67  SI4464  [SI4464]
U68  SHT40-AD1B-R2  [SHT40]
U69  RY8310  [SOT23-6]
U70  RP2040  [QFN40P700X700X90-57N]
U71  RFM98PW  [RFM98PW]
U72  RFM-0505S  [RFM0505S]
U73  RASPBERRY_PICOTH  [PICO-PKG-TH]
U74  PE42441C-Z  [QFN32-55]
U75  PDSE1-S5-S9-S  [PDSE1-S]
U76  PDSE1-S5-S5-S  [PDSE1-S]
U77  PCM1681PWPR  [TSSOP28-POWER]
U78  P78E05-1000  [P78E05-1000]
U79  OPA2320AIDGKR  [8-VSSOP]
U80  OPA211AIDR  [SOIC8]
U81  NE555PSR  [SOIC8]
U82  NCV5183DR2G  [SOIC8]
U83  NCP5901BDR2G  [SOIC8]
U84  NCP781BMNADJTAGOSCT-ND  [6DFN]
U85  NCP508SQ28T1G  [SOT-353]
U86  MTI-7-T  [MTI-1S]
U87  MPQ4436GRE-AEC1-Z  [MPQ-QFN-20-4X4]
U88  MP86952  [MP86952]
U89  MP5515  [MP5515]
U90  MP3423  [QFN14_MPS]
U91  MIC28516T-E/PHA  [MIC28516]
U92  MIC7221YM5-TR  [SOT23-5]
U93  MIC4604YM-TR  [SOIC8]
U94  12V  MIC2920A-12WS  [SOT223]
U95  MIC2288  [SOT23-5]
U96  MIC2176-1YMM  [MSOP10]
U97  MIC842LYC5-TR  [SC-70-5]
U98  ME6211C12M5G-N  [SOT23-5]
U99  MCP73832T-5ACI/OT  [SOT23-5]
U100  MCP73811T-420I/OT  [SOT23-5]
U101  MCP73114-0NSI/MF  [10DFN]
U102  MCP23017  [SSOP28]
U103  MCP9700  [SOT23-3]
U104  MCP6561T-E/OTVAO  [SOT23-5]
U105  MCP6549-I/ST  [TSSOP14]
U106  MCP6542T-I/SN  [SOIC8]
U107  MCP4725A1T-E/CH  [SOT23-6]
U108  MCP1702T-5002E/CB  [SOT23-3_CENTERED]
U109  MCP1665T-E/MRA  [2X2VQFN_MCP1665]
U110  MCP1632-BAE/MS  [MSOP-8]
U111  MCP1407-E/SN  [SOIC8]
U112  MCP6L01T-E/OT  [SOT23-5]
U113  MC14044BDR2G  [SO16]
U114  MC14043BDR2G  [SO16]
U115  MC74LVX08DTR2G  [SOP65P640X120-14N]
U116  MAX9107  [SOIC8]
U117  MAX9095ASD+  [SO14]
U118  MAX5084ATT+T  [6DFN-EP]
U119  MAX3232ECDR  [SOIC16_TI]
U120  MAX2680  MAX2680AUT+T  [SOT23-6]
U121  MAX2671EUT+T  [SOT23-6]
U122  MAX2663  MAX2663EUT+T  [SOT23-6]
U123  MAX232  [SOIC16]
U124  MAX-M8Q-0  [MAX-M8]
U125  LTV827S-TA1  [8SMD]
U126  LTV-816S  [LTV-816S]
U127  LTC6993CS6-1#TRMPBF  [SOT23-6]
U128  LTC6992CS6-1#TRMPBF  [SOT23-6]
U129  LTC6990CS6#TRMPBF  [SOT23-6]
U130  LTC4365  [TSOT-23-8]
U131  LT8410IDC#TRMPBF  [8DFN]
U132  LT6654BHS6-2.5#TRMPBF  [SOT23-6]
U133  LT3088EDD#PBF  [8DFN_LT]
U134  LT3080  [SOT223]
U135  LT3012EFETRPBFTSSOP-16_FE/BB_LIT-M  [TSSOP-16_FE/BB_LIT-M]
U136  LT1678  [SOIC8]
U137  LT1054  [SOP16]
U138  LP28013A  [10DFN]
U139  LMV7219M5X  [SOT23-6]
U140  LMV321IDBVR  [SOT23-5]
U141  LMT87LPG  [TO-92]
U142  LMR38020SDDAR  [SOIC8_TP_TI]
U143  LMP2231  [SOT23-5]
U144  LMC7660  [SOP8]
U145  LMC662CN/NOPB  [110-87-308-41-105191]
U146  LMC662CMX/NOPB  [SOIC8]
U147  LMC555CMM/NOPB  [8-VSSOP]
U148  LM46002AQPWPRQ1  [TSSOP16-POWER]
U149  LM25116MHX/NOPB  [HTSSOP20]
U150  LM7301  [SOT23-5]
U151  LM5155  [12-WSON]
U152  LM5134-SOT  [SOT23-6]
U153  LM5102MM/NOPB  [VSSOP10]
U154  LM4040DYM3-2.5-TR  [SOT23-3]
U155  LAN9512  [64QFN_9X9]
U156  LAN8742A-CZ-TR  [QFN24-44]
U157  L6491  [SO14]
U158  L5150BNTR  [SOT223]
U159  L4931  [SOP8]
U160  L78M05ABDT-TR  [TO-252]
U161  K78U05-500R3  [K78U05-500R3]
U162  ISO1640BDR  [SOIC8]
U163  ISL83490IBZ-T  [SOIC8]
U164  1.25V  ISL21080DIH312Z-TK  [SOT23-3]
U165  IRS2304SPBF  [SOIC8]
U166  IRS2186  [SOIC8]
U167  IRM-05-5  [IRM-05-5]
U168  INA240A3PW  [TSSOP8]
U169  INA210CIDCKR  [SC-70]
U170  INA195  INA195AIDBVR  [SOT23-5]
U171  INA181A3IDBVR  [SOT23-6]
U172  INA180A3IDBVR  [SOT23-5]
U173  HTCC-AB01  [HTCC-AB01]
U174  HMC544A  [SOT23-6]
U175  HMC385  HMC385LP4E  [QFN24-55]
U176  HELTEC_WIFI_LORA_32_V3  [HELTEC_WIFI_LORA_32_V3]
U177  HEF4052B  [SO16]
U178  HD3SS3412ARUAT  [WQFN42]
U179  HCF4010YM013TR  [SO16]
U180  GVA-84+  [SOT-89A]
U181  FT232RL  [SSOP28]
U182  FM2113  [SOT23-6]
U183  FAN3180  [SOT23-5]
U184  FAN3111ESX  [SOT23-5]
U185  EL5171  [SOIC8]
U186  DS1100Z-500  [SOIC8]
U187  DS18S20  [TO92]
U188  DRV8231ADDAR  [SOIC8_TP]
U189  DP83822IRHBR  [QFN32-55_TI]
U190  DP83TD510ERHBR  [QFN32-55_TI]
U191  DAC5571IDBVR  [SOT23-6]
U192  48MHZ  COM13025-48.000-T-TR  [4SMD]
U193  CO32H4-25.000-33GDTST  [3.2X2.5_4SMD]
U194  CM108  [LQFP48]
U195  CD40257  [SOIC16]
U196  CD74HC4017M96  [SOIC16_TI]
U197  CBTL02042ABQ,115  [DHVQFN20]
U198  BQ7790512PWR  [TSSOP20]
U199  BQ24616  [QFN24-44_TI]
U200  BQ24171  [P-VQFN-N24]
U201  BNO080  [BNO080]
U202  BMP280  [BME280]
U203  BGU8051  [SOT1327-1]
U204  BGU6102  BGU6102,147  [6-XFDFN]
U205  BGB741L7ESDE6327XTSA1  [PG-TSLP-7-1]
U206  BGA2869,115  [SOT-363]
U207  BGA2866  BGA2866,115  [SOT-363]
U208  BGA427H6327XTSA1  [SOT-343]
U209  BD9C401EFJ-E2  [SOIC8_TP]
U210  B39921B2672P810  [B2672]
U211  B39431B3710U410  [6SMD_SAW]
U212  AX5043  [QFN28-55]
U213  ATTINY85V-10SUR  [SOIC8]
U214  ATA6561-GAQW-N  [SOIC8]
U215  AT2659  [6DFN-1X1.6]
U216  AP65550  AP65550SP-13  [SOIC8_TP]
U217  AP9211SA  [AP9211SA]
U218  AP2114H-3.3  [SOT223]
U219  AP2114H-2.5  [SOT223]
U220  AP2114H-1.8  [SOT223]
U221  AOZ128  [SOIC8_TP]
U222  AMS1117-3.3  [SOT223]
U223  AG1170  [AG1170S]
U224  ADS1115IDGSR  [VSSOP10]
U225  ADP7142AUJZ-3.3-R7  [SOT23-5]
U226  ADG812YRUZ-REEL7  [TSSOP16]
U227  ADF4351  [ADF4351]
U228  ADF4118  ADF4118BRUZ  [TSSOP16]
U229  AD8306  [SO16]
U230  ACS781KLRTR-150B-T  [7POWERSMD]
U231  ACS711ELCTR-25AB-T  [SOIC8]
U232  ACS711ELCTR-12AB-T  [SOIC8]
U233  ACPL-782T-300E  [8SMD]
U234  0026605020  [3.96MM]
U235  74VHC4040FT  [TSSOP16]
U236  74LVCH2T45DC,125  [VSSOP8]
U237  74LVC4245A  [SOIC24]
U238  74HC4051D,653  [SO16]
U239  74AHC14PW,112  [TSSOP14]
U240  000  [SO16]
U$1  ZF43610  [TRANSFORMER]
U$2  XT30PW-F  [XT30PW-F]
U$3  WA-T247-101E  [WA-T247-101E]
U$4  VERT-55351  [VERT-55351]
U$5  UA78M33CKVURG3  [TO-252]
U$6  TRF37D73IDSGT  [8-WFDFN]
U$7  TP65H035WS  [TO-247]
U$8  TOROID2  [INDUCTOR4]
U$9  TOROID1  [INDUCTOR3]
U$10  TDA21490  [MP86952]
U$11  STW40N65M2  [TO-247]
U$12  SPU01M-05  [SPU01M-05]
U$13  SP1312/S  [SP1312/S]
U$14  SIP32408DNP-T1-GE4  [TDFN4]
U$15  PLUG  [738W-X2/01]
U$16  PINHD20  [1X20]
U$17  PA1005.100NLT  [PA1005.100NLT]
U$18  OLED  [OLED]
U$19  MC3417  [DIP_SOCKET_16]
U$20  LM25037  [TSSOP16]
U$21  LM5134  [WSON]
U$22  HMC313E  [SOT23-6]
U$23  EPC2033  [EPC2033]
U$24  25MHz  ECS-250-18-36B-CKY-TR  [4SMD]
U$25  DS02C-254-1L-04BE  [4DIP_RA]
U$26  CSAC  [CSAC]
U$27  COUPLED_INDUCTOR2  [C055071-COUPLED2]
U$28  COUPLED_INDUCTOR  [C055071-COUPLED3]
U$29  CMZ5951CTR13  [DO-214AC]
U$30  BGA6589  BGA6589,135  [SOT-89A]
U$31  B38G3RGB-10D0003H2U1930  [1616]
U$32  ADA4891-2ARZ-R7  [SOIC8]
U$33  AD8317  [AD8317]
U$34  74439358010  [74439358010]
U$35  1841513  [1841513]
U$36  100UH41A  [18MMINDUCTOR2]
U$37  100UH4A  [18MMINDUCTOR]
U$38  10AWG  [10AWG]
U$39  3:1TRANSFORMER  [TRANSFORMER2]
U$40  .42UH  [MCP0740]
V1  IV-6  [IV-6]
VR1  ST4ETA104  [SMDPOT]
VR2  ST4ETA102  [SMDPOT]
VR3  PTV09A-4225F-B104  [PTV09]
VR4  P160KN-0QC15B500K  [P160]
VR5  3224G-1-104E  [3224G]
X1  TA0862A  [TA0862A]
X2  TA0289A  [TA0289A]
X3  SIT2024AA-S2-XXE-25.000000E  [SOT23-5]
X4  SIT2024AA-S2-XXE-8.000000E  [SOT23-5]
X5  RTX-2520AF333-S-32.000-TR  [4SMD]
X6  RTX-2520AF3F-S-10.000-TR  [RTX-2520]
X7  NX2016SA-32M-EXS00A-CS06465  [NX2016SA-32M-EXS00A-CS06465]
X8  32.7680KHZ  FC-13532.7680KA-AC0  [2SMD_CRYSTAL]
X9  F6HH2G350EH75-J  [EH75]
X10  DSC1124DI5-390.0250T  [DSC1124]
X11  30 MHz  ABM8-30.000MHZ-10-1-U-T  [4SMD]
X12  12MHz  ABLS-12.000MHZ-B2-T  [HC-49/US]
X13  8MHz  ABLS-8.000MHZ-B4-T  [HC-49/US]
X14  6MHz  ABLS-6.000MHZ-20-B-3-H-T  [HC-49/US]
X15  4MHz  ABLS-4.000MHZ-B2-T  [HC-49/US]
Z1  ADE-25MH+  [CD]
